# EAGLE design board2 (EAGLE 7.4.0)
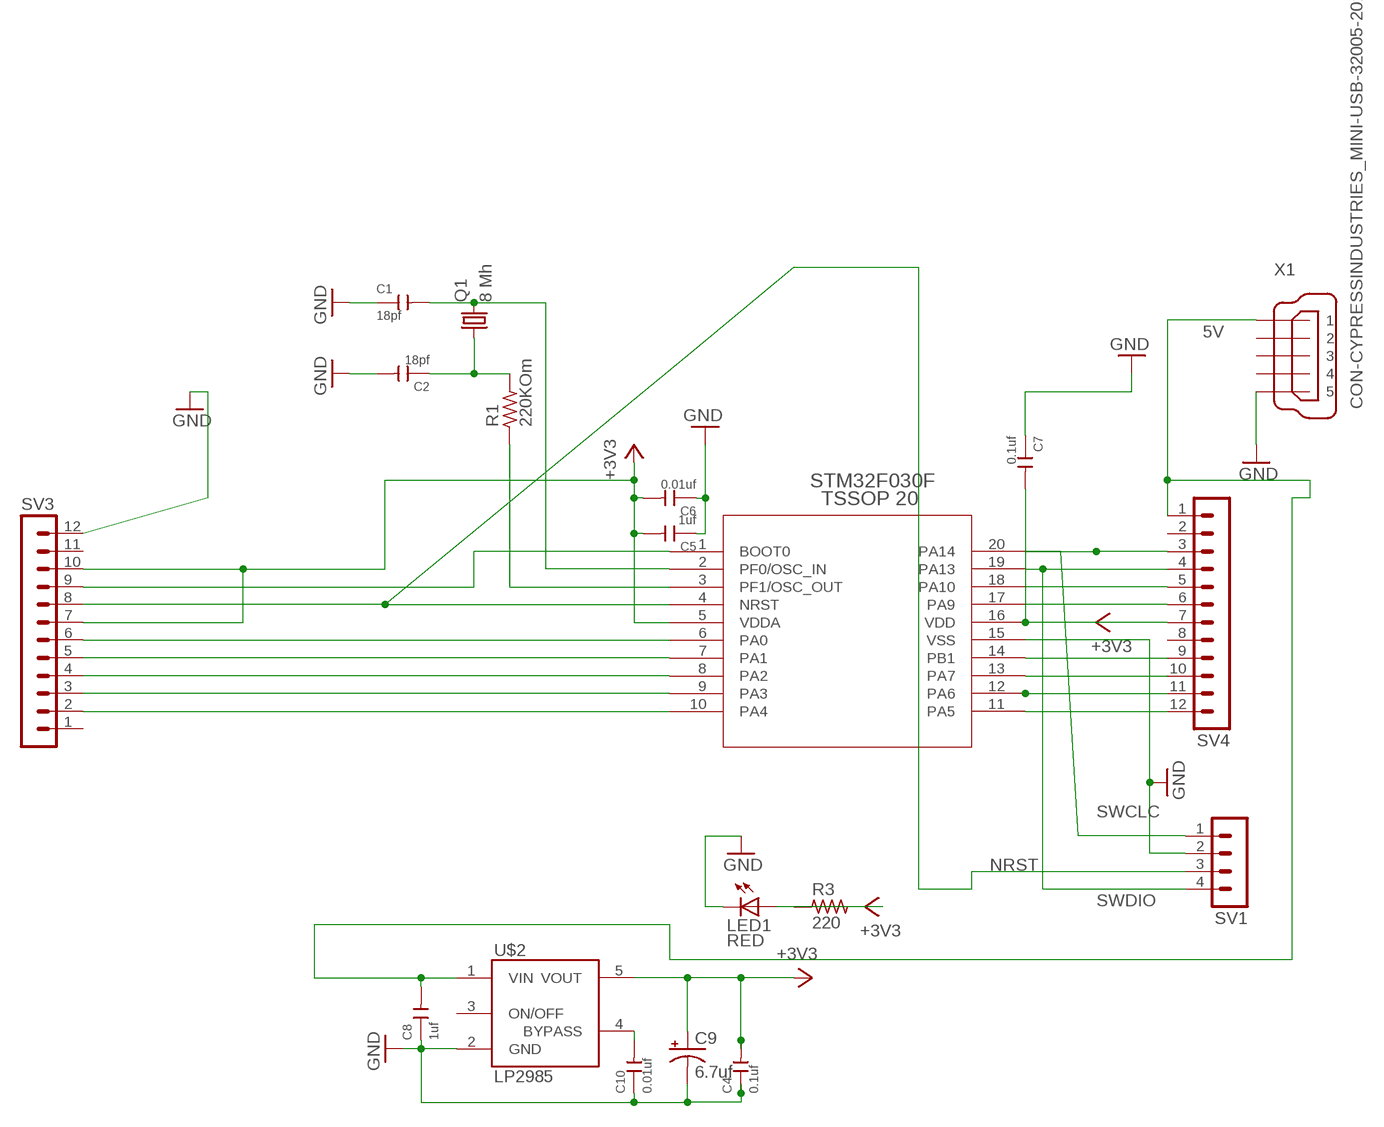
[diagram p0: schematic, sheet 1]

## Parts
C1  18pf  CERAMIC-10UF-25V-10%-X5R(1206)  [C1206]
C2  18pf  CERAMIC-10UF-25V-10%-X5R(1206)  [C1206]
C4  0.1uf  CERAMIC-4.7UF-50V-10%-X5R(1206)  [C1206]
C5  1uf  CERAMIC-4.7UF-50V-10%-X5R(1206)  [C1206]
C6  0.01uf  CERAMIC-4.7UF-50V-10%-X5R(1206)  [C1206]
C7  0.1uf  CERAMIC-4.7UF-50V-10%-X5R(1206)  [C1206]
C8  1uf  CERAMIC-4.7UF-50V-10%-X5R(1206)  [C1206]
C9  6.7uf  CAP_POL7343  [EIA7343]
C10  0.01uf  CERAMIC-4.7UF-50V-10%-X5R(1206)  [C1206]
LED1  RED  STM32F050F-BASE_LEDCHIPLED_1206  [STM32F050F-BASE_CHIPLED_1206]
Q1  8 Mh  CRYSTALHC49S  [HC49/S]
R1  220KOm  STM32F050F-BASE_R_1206  [STM32F050F-BASE_R1206]
R3  220  STM32F050F-BASE_R_1206  [STM32F050F-BASE_R1206]
SV1  MA04-1  [MA04-1]
SV3  MA12-1  [MA12-1]
SV4  MA12-1  [MA12-1]
U$1  STM32F050F-BASE_STM32F050F4P6  [STM32F050F-BASE_TSSOP20]
U$2  LP2985_LP2985AIM5-3.3  [LP2985_SOT25]
X1  CON-CYPRESSINDUSTRIES_MINI-USB-32005-201  [CON-CYPRESSINDUSTRIES_32005-201]

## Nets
5V: C8.2 SV4.1 U$2.1(VIN) X1.1
+3V3: C4.2 C5.2 C6.2 C7.2 C9.A(+) R3.1 SV3.7 SV3.10 SV4.7 U$1.5(VDDA) U$1.16(VDD) U$2.5(VOUT)
BYPASS: C10.2 U$2.4(BYPASS)
GND: C1.1 C2.2 C4.1 C5.1 C6.1 C7.1 C8.1 C9.C(-) C10.1 LED1.C SV1.2 SV3.12 U$1.15(VSS) U$2.2(GND) X1.5
N$2: LED1.A R3.2
N$3: SV4.12 U$1.11(PA5)
N$4: SV3.2 U$1.10(PA4)
N$5: SV4.11 U$1.12(PA6)
N$6: SV4.10 U$1.13(PA7)
N$7: SV4.9 U$1.14(PB1)
N$8: SV4.6 U$1.17(PA9)
N$9: SV4.5 U$1.18(PA10)
N$10: SV3.3 U$1.9(PA3)
N$12: SV3.4 U$1.8(PA2)
N$13: C2.1 Q1.1 R1.2
N$14: SV3.5 U$1.7(PA1)
N$15: SV3.6 U$1.6(PA0)
N$16: SV3.9 U$1.1(BOOT0)
N$21: R1.1 U$1.3(PF1/OSC_OUT)
N$25: C1.2 Q1.2 U$1.2(PF0/OSC_IN)
NRST: SV1.3 SV3.8 U$1.4(NRST)
SWCLC: SV1.1 SV4.3 U$1.20(PA14)
SWDIO: SV1.4 SV4.4 U$1.19(PA13)
Unconnected: SV3.1 SV3.11 SV4.2 SV4.8 U$2.3(ON/OFF) X1.2 X1.3 X1.4

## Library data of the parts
C1 C2 = Seeed-OPL-Capacitor:CERAMIC-10UF-25V-10%-X5R(1206): 302010181; MPN: CC1206KKX5R8BB106; VALUE: 10uf
C4-C8 C10 = Seeed-OPL-Capacitor:CERAMIC-4.7UF-50V-10%-X5R(1206): 302010243; MPN: CC1206KKX5R9BB475; VALUE: 4.7uf
C9 = SparkFun-Capacitors:CAP_POL: Capacitor Polarized; PROD_ID: CAP-08702
LED1 = clockclock1:STM32F050F-BASE_LED: LED
Q1 = crystal:CRYSTAL: CRYSTAL; OC_FARNELL: 1667008; OC_NEWARK: unknown
R1 R3 = clockclock1:STM32F050F-BASE_R_: RESISTOR
SV1 = con-lstb:MA04-1: PIN HEADER; OC_FARNELL: unknown; OC_NEWARK: unknown
SV3 SV4 = con-lstb:MA12-1: PIN HEADER; OC_FARNELL: unknown; OC_NEWARK: unknown
U$1 = clockclock1:STM32F050F-BASE_STM32F050F4P6: STM32F050F4P6
U$2 = clockclock1:LP2985_LP2985: LP2985-N Micropower 150 mA Low-Noise Ultra Low-Dropout Regulator
X1 = clockclock1:CON-CYPRESSINDUSTRIES_MINI-USB-: MINI USB-B Conector Source: www.cypressindustries.com; OC_FARNELL: unknown; OC_NEWARK: unknown

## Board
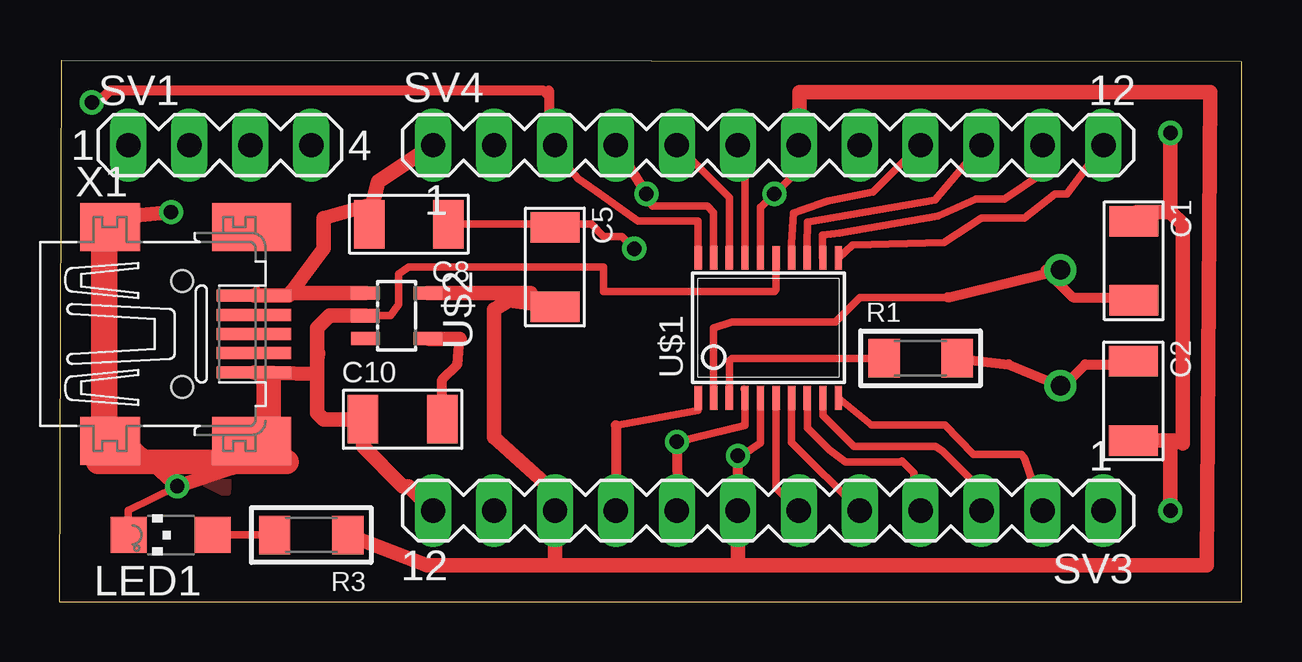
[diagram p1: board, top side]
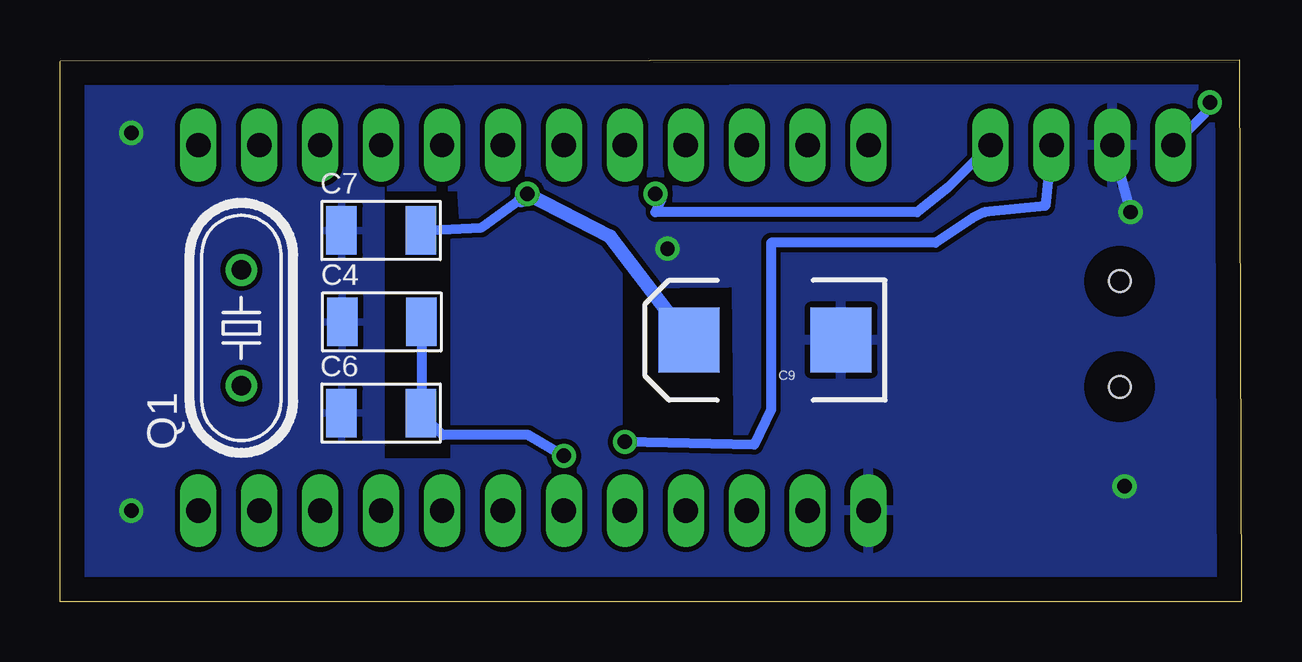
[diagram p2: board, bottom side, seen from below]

Size 49.26 x 22.6 mm. Coordinates in mm from the lower left corner, seen from the top.
Outline: 49.26,22.53 49.26,0 0,0 0.08,22.6 49.25,22.55
Copper layers (1*16): Top 0.035mm / dielectric 1.5mm / Bottom 0.035mm
Design rules "default": minimum track width 10mil, minimum drill 24mil, track to track 8mil, track to pad 8mil, pad to pad 8mil, via to via 8mil, smd to smd 8mil, copper to edge 40mil, drill to drill 8mil, minimum pad ring 10mil, minimum via ring 8mil, stop-mask expansion 4mil, vias tented up to drill 0mil, thermal gap 10mil

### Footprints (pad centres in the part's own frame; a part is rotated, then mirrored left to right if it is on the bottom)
C1206 = smd 1.27 x 2.032: 1 -1.651,0; 2 1.651,0
EIA7343 = smd 2.55 x 2.7: A 3.17,0; C -3.17,0
STM32F050F-BASE_CHIPLED_1206 = smd 1.5 x 1.5: A 0,-1.75; C 0,1.75
HC49/S = drill 0.813: 1 -2.413,0; 2 2.413,0
STM32F050F-BASE_R1206 = smd 1.3 x 1.6: 1 -1.524,0; 2 1.524,0
MA04-1 = drill 1.016 long: 1 -3.81,0; 2 -1.27,0; 3 1.27,0; 4 3.81,0
MA12-1 = drill 1.016 long: 1 -13.97,0; 2 -11.43,0; 3 -8.89,0; 4 -6.35,0; 5 -3.81,0; 6 -1.27,0; 7 1.27,0; 8 3.81,0; 9 6.35,0; 10 8.89,0; 11 11.43,0; 12 13.97,0
STM32F050F-BASE_TSSOP20 = smd 0.305 x 0.991: 1 -2.925,-2.918; 2 -2.275,-2.918; 3 -1.625,-2.918; 4 -0.975,-2.918; 5 -0.325,-2.918; 6 0.325,-2.918; 7 0.975,-2.918; 8 1.625,-2.918; 9 2.275,-2.918; 10 2.925,-2.918; 11 2.925,2.918; 12 2.275,2.918; 13 1.625,2.918; 14 0.975,2.918; 15 0.325,2.918; 16 -0.325,2.918; 17 -0.975,2.918; 18 -1.625,2.918; 19 -2.275,2.918; 20 -2.925,2.918
LP2985_SOT25 = smd 0.55 x 1.2: 1 -0.95,-1.3; 2 0,-1.3; 3 0.95,-1.3; 4 0.95,1.3; 5 -0.95,1.3
CON-CYPRESSINDUSTRIES_32005-201 = smd 3.1 x 0.5: 1 3,1.6; 2 3,0.8; 3 3,0; 4 3,-0.8; 5 3,-1.6 | smd 2.5 x 2: M1 -3,-4.45; M2 -3,4.45 | smd 3.3 x 2: M3 2.9,4.45; M4 2.9,-4.45 | hole 0.9: 0,2.2; 0,-2.2

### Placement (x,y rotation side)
C1  44.76,14.22 270 top
C2  44.74,8.38 270 top
C4  35.84,11.68 0 bottom
C5  20.63,13.96 270 top
C6  35.87,7.87 0 bottom
C7  35.87,15.49 0 bottom
C8  14.54,15.75 180 top
C9  19.87,10.92 180 bottom
C10  14.28,7.62 0 top
LED1  4.62,2.79 90 top
Q1  41.7,11.43 90 bottom
R1  35.87,10.16 0 top
R3  10.47,2.79 180 top
SV1  6.66,19.05 0 top
SV3  29.52,3.81 180 top
SV4  29.52,19.05 0 top
U$1  29.52,11.43 0 top
U$2  14.03,11.94 270 top
X1  5.09,11.18 0 top

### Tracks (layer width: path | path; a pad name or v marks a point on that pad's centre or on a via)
5V
  Top 0.305: 8.19,13.03 X1.1
  Top 0.406: 12.76,16.51 12.63,16.51 C8.2
  Top 0.61: X1.1 9.53,12.78 9.68,12.98 | 9.68,12.98 10.98,14.73 10.98,16 12.76,16.51 13.01,16.51 13.27,17.53 SV4.1 | U$2.1 9.68,12.89 9.68,12.98
+3V3  (via drill 0.6)
  Top 0.305: U$1.5 29.19,6.63 28.41,6.1 | 28.25,5.08 SV3.7 | U$1.16 29.19,16.46 29.22,16.46 v29.78,17.02 30.79,18.03 SV4.7 30.79,18.8
  Top 0.406: 28.25,5.08 v28.25,6.1 28.41,6.1 | 19.62,12.89 C5.2
  Top 0.61: 11.87,2.92 R3.1 15.3,1.52 20.63,1.52 | 20.63,1.52 SV3.10 20.63,4.57 18.09,6.86 18.09,12.19 18.72,12.56 C5.2 | 20.63,1.52 28.25,1.52 | 28.25,1.52 SV3.7 | 28.25,1.52 47.81,1.52 47.94,21.26 30.82,21.26 SV4.7 | U$2.5 19.62,12.89
  Bottom 0.406: C7.2 31.68,15.62 v29.78,17.02 | v28.25,6.1 29.73,6.96 33.31,6.96 C6.2 34.19,7.91 C4.2
  Bottom 0.61: C9.A 26.32,15.24 v29.78,17.02 30.03,16.76
BYPASS
  Top 0.406: C10.2 15.94,9.27 16.57,9.91 16.65,10.97 | 15.4,10.97 U$2.4
  Top 0.61: 16.65,10.97 15.4,10.97
GND  (via drill 0.6)
  Top 0.305: v4.89,4.83 2.85,3.81 LED1.C | 46.67,10.03 46.8,9.91 | 44.88,16.26 C1.1 | U$1.15 29.85,13.03 29.78,12.95 22.67,12.95 22.67,13.97 14.54,13.97 14.11,13.67 14.11,12.39 13.78,11.94 U$2.2 | C5.1 20.5,15.75 C8.1 22.16,15.75 22.67,15.24 23.43,15.24 v23.94,14.73
  Top 0.61: 8.7,6.35 7.17,5.59 v4.89,4.83 2.09,7.37 2.09,16 v4.63,16.26 | 44.88,16.26 46.29,16.26 | 46.29,16.26 46.8,15.75 46.8,9.91 46.8,6.6 46.42,6.73 46.29,6.73 | C2.2 46.29,6.73 | v46.29,3.81 46.29,6.73 | v46.29,19.56 46.29,16.26 | 10.73,9.4 10.73,7.87 10.98,7.62 C10.1 12.63,6.48 14.28,4.83 14.54,4.83 SV3.12 | 10.73,9.4 10.73,10.16 | 10.73,10.16 10.73,11.43 11.24,11.94 U$2.2 | 10.77,10.38 10.73,10.16 | X1.5 10.65,9.5 10.73,9.4
  Top 1.016: 8.7,9.17 8.7,6.35
  Bottom 0.406: v4.63,16.26 SV1.2
  pour Top: 6.92,4.57 7.17,7.11 1.33,7.37
  pour Bottom: 0.57,22.1 0.57,0.51 20.89,0.51 21.14,22.1
  pour Bottom: 35.87,22.35 35.87,5.84 32.83,5.84 32.83,13.46 32.83,13.72 32.83,16.76 32.57,16.76 32.57,17.53 25.97,17.53 25.97,6.1 20.38,6.1 20.38,0.51 35.87,0.51 49.08,0.25 49.08,22.1
  pour Bottom: 1.08,21.59 1.08,13.46 25.46,13.21 25.46,14.22 25.97,14.22 25.97,13.46 32.32,13.46 32.57,17.27 36.38,17.27 36.38,21.34 35.87,21.34 35.87,21.59
N$2
  Top 0.305: R3.2 LED1.A
N$3
  Top 0.305: U$1.11 33.04,14.88 36.84,14.98 38.41,16.01 40.18,16.01 40.19,16 41.46,17.02 41.97,17.02 SV4.12
N$4
  Top 0.305: U$1.10 33.82,7.39 36.88,7.39 38.08,6.14 40.07,6.14 40.19,6.01 SV3.2
N$5
  Top 0.305: SV4.11 40.98,17.89 39.37,16.79 38.18,16.79 36.58,16.09 32.48,15.39 31.78,15.29 31.78,14.36 U$1.12
N$6
  Top 0.305: U$1.13 31.14,14.84 31.16,15.84 36.47,16.75 SV4.10
N$7
  Top 0.254: 35.87,19 SV4.9
  Top 0.305: U$1.14 30.5,14.95 30.56,16.21 31.98,16.71 33.87,17.09 33.88,17.09 35.84,19.05 SV4.9
N$8
  Top 0.305: SV4.6 28.55,18.75 U$1.17
N$9
  Top 0.305: SV4.5 27.9,16.86 U$1.18
N$10
  Top 0.305: U$1.9 31.8,7.77 33.08,6.49 36.48,6.49 36.78,6.29 38.28,4.79 38.28,3.94 SV3.3
N$12
  Top 0.305: U$1.8 31.15,7.27 32.06,6.35 32.73,5.85 35.04,5.85 35.08,5.89 35.58,5.39 35.58,4.1 SV3.4
N$13
  Top 0.406: R1.2 39.54,9.91 Q1.1 41.84,9.02 42.73,9.91 44.61,9.91 C2.1
N$14
  Top 0.305: SV3.5 30.5,6.65 U$1.7
N$15
  Top 0.305: SV3.6 29.85,4.76 U$1.6
N$16
  Top 0.305: U$1.1 26.6,8 23.17,7.37
  Top 0.406: 23.17,7.37 SV3.9
N$21
  Top 0.305: U$1.3 27.9,10.06 28,10.16 R1.1
N$25
  Top 0.305: U$1.2 27.24,11.43 28,11.68 32.32,11.68 33.33,12.7 37,12.7
  Top 0.406: 37,12.7 Q1.2 41.08,13.84 42.22,12.7 44.63,12.7 C1.2
N$27
  Top 0.61: 1.58,15.75 1.58,5.84
  Top 1.016: 1.58,5.84 9.46,5.84
NRST  (via drill 0.6)
  Top 0.305: 28.51,8.89 28.55,8.85 U$1.4 28.56,7.37 v25.71,6.68 | 25.74,4.14 SV3.8 25.74,3.84
  Top 0.406: v25.71,6.68 25.74,4.14
  Bottom 0.406: SV1.3 8.19,16.51 10.73,16.26 11.24,16 12.76,14.99 19.62,14.99 19.62,8.03 20.32,6.56 v25.71,6.68
SWCLC  (via drill 0.6)
  Top 0.305: U$1.20 26.58,14.36 26.58,15.89 24.08,15.89 22.34,17.14 21.6,17.64 20.89,18.46 SV4.3
  Top 0.406: 20.38,21.34 20.38,21.08 | 20.38,21.08 20.38,19.3 SV4.3 | v1.33,20.83 1.58,20.83 2.09,21.34 20.13,21.34 20.38,21.08
  Bottom 0.406: v1.33,20.83 1.58,20.32 SV1.1
SWDIO  (via drill 0.6)
  Top 0.305: SV4.4 24.7,16.51 26.98,16.51 27.25,16.25 U$1.19
  Top 0.406: v24.44,17.02 SV4.4
  Bottom 0.406: SV1.4 12.25,17.27 13.52,16.26 24.44,16.26 24.19,16.76 v24.44,17.02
